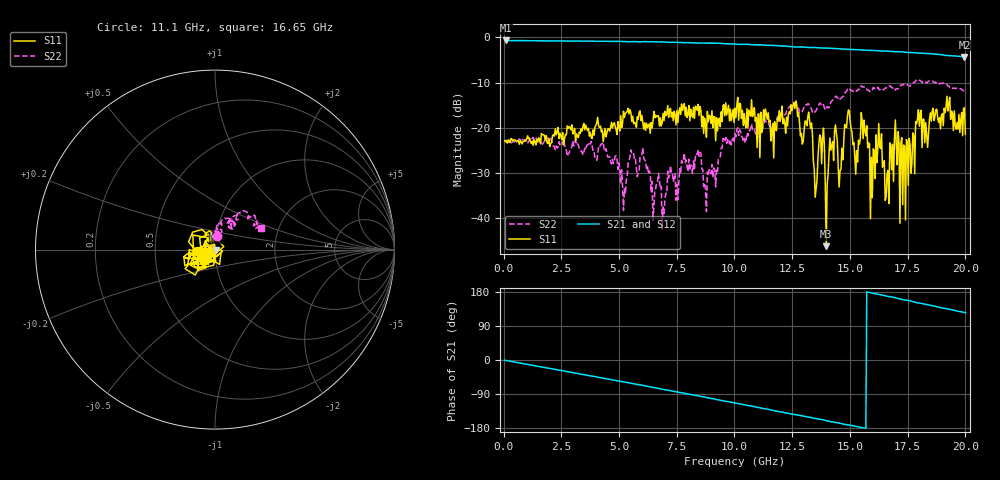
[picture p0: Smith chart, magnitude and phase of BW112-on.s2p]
!  2-Port S-parameters saved by WinCal
! VAR MeasName=S-Parameters (CALIBRATED_DATA) read from VNA (E8364A)
! VAR MeasDate=10/8/2010 5:31:40 PM
! VAR NAME=3(40)-on
! VAR FILENAME=3(40)-on.s2p
! VAR DATE=10/8/2010 5:31:40 PM
! VAR PHYS_PORTS=1,2
# Hz S RI R 50
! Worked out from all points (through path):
!   501 points, 45 MHz to 20 GHz, reference 50 ohm
!   highest |S21| = -0.69 dB at 84.91 MHz (marker M1); lowest = -4.3 dB at 19.96 GHz (marker M2)
!   group delay of S21, straight-line fit = 32.5 ps
!   lowest |S11| = -46.1 dB at 13.97 GHz (marker M3), VSWR 1.01, Z = 50.5 - j0.0418 ohm
!   |S11| at or under -10 dB: start of sweep to end of sweep
!   |S22| runs from -42.4 to -9.3 dB; largest |S21 - S12| = 0.0079
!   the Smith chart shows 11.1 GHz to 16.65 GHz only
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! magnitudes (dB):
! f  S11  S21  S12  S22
! 45 MHz  -22.9  -0.7  -0.7  -23.0
! 84.91 MHz  -22.7  -0.7  -0.7  -23.1
! 3.397 GHz  -20.7  -0.9  -0.9  -25.2
! 6.71 GHz  -17.3  -1.0  -1.0  -30.0
! 6.949 GHz  -18.4  -1.0  -1.1  -38.9
! 8.466 GHz  -17.3  -1.2  -1.3  -26.3
! 8.745 GHz  -19.2  -1.3  -1.3  -33.6
! 10.02 GHz  -15.6  -1.5  -1.5  -21.3
! 12.62 GHz  -15.7  -2.1  -2.1  -14.6
! 13.37 GHz  -21.2  -2.3  -2.3  -16.5
! 13.49 GHz  -35.3  -2.3  -2.3  -16.4
! 13.81 GHz  -22.4  -2.3  -2.4  -14.6
! 13.97 GHz  -46.1  -2.4  -2.4  -15.6
! 14.93 GHz  -16.0  -2.6  -2.7  -11.3
! 15.25 GHz  -30.2  -2.7  -2.7  -12.0
! 15.57 GHz  -22.4  -2.8  -2.8  -11.0
! 15.89 GHz  -40.1  -2.9  -2.9  -11.7
! 16.69 GHz  -36.7  -3.1  -3.1  -10.8
! 17.37 GHz  -24.1  -3.3  -3.3  -10.3
! 18 GHz  -19.6  -3.5  -3.5  -9.5
! 19.96 GHz  -15.5  -4.3  -4.4  -12.3
! 20 GHz  -21.4  -4.3  -4.3  -12.2
